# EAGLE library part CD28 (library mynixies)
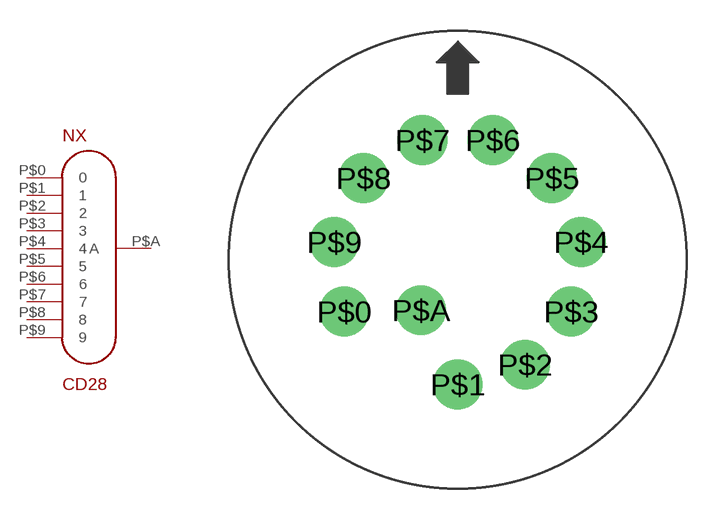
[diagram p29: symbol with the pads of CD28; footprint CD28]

Designator prefix NX

## CD28  [CD28]
P$0  0  pas
P$1  1  pas
P$2  2  pas
P$3  3  pas
P$4  4  pas
P$5  5  pas
P$6  6  pas
P$7  7  pas
P$8  8  pas
P$9  9  pas
P$A  A  pas

## Footprint CD28 (pad centres in mm)
drill 1.6: P$0 -5.457,-2.495; P$1 0,-6; P$2 3.244,-5.047; P$3 5.458,-2.492; P$4 5.939,0.855; P$5 4.534,3.93; P$6 1.689,5.757; P$7 -1.692,5.756; P$8 -4.536,3.928; P$9 -5.939,0.852; P$A -1.763,-2.427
